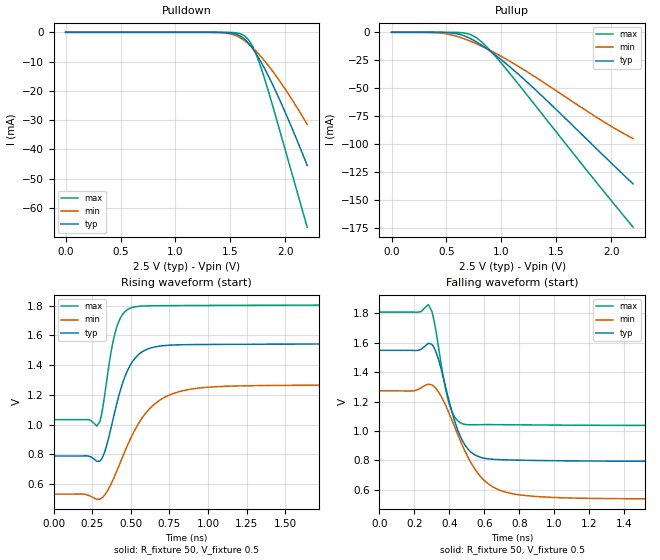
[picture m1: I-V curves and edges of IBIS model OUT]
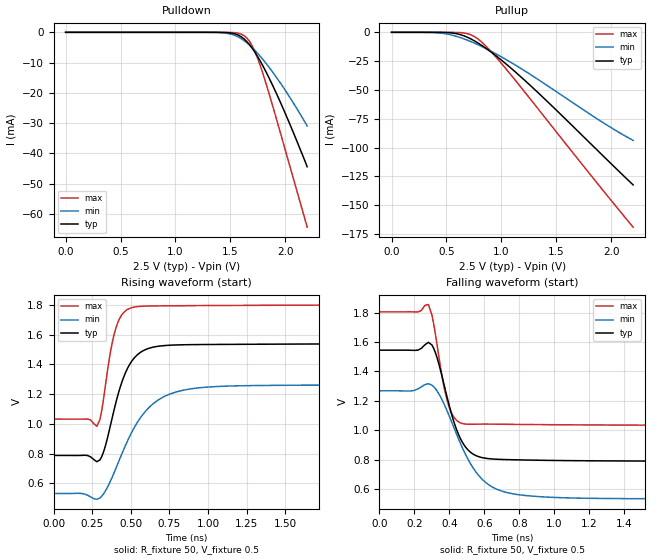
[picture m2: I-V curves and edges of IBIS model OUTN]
|   IBIS File of SG2520EGN D
|   LV-PECL, Vcc=2.5V, fo<=212.5MHz
[IBIS Ver]   3.2
[File Name]   sg2520egn_25v.ibs
[File Rev]   1.0
[Date]   Sep. 2, 2020
[Source]
[Notes]
Created by Minoru Kozaki
[Disclaimer]
Seiko Epson Corporation makes no warranty with respect to the
information contained herein.
[Copyright]
Copyright(C) 2020, Seiko Epson Corporation. All rights reserved.
|   Component
[Component]   SG2520EGN
[Manufacturer]  Seiko Epson Corporation
[Package]
R_pkg   17.7m   NA   NA
L_pkg   235p   NA   NA
C_pkg   208f   NA   NA
[Pin]   signal_name   model_name   R_pin   L_pin   C_pin
1   OE/ST   NC
2   NC   NC
3   GND   GND
4   OUT   OUT   17.7m   235p   208f
5   OUTN   OUTN   10.4m   129p   221f
6   VCC   POWER
[Diff Pin] inv_pin  vdiff  tdelay_typ
4   5   0   0
| Models and submodels in the file (2): OUT (Output_ECL), OUTN (Output_ECL)
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|   Model OUT
[Model]   OUT
Model_type   Output_ECL
Polarity   Non-Inverting
Vref = 0.5
Vmeas = 1.166
Rref = 50
Cref = 0
C_comp   0.5p   0.5p   0.5p
[Temperature Range]   25   105   -40
[Voltage Range]   2.5   2.25   2.75
[Pullup Reference]   2.5   2.25   2.75
[Pulldown Reference]   2.5   2.25   2.75
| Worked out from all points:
|   falling waveform, R_fixture 50, V_fixture 0.5: 20-80 % time 113ps typ, 187ps min, 71.3ps max; typ from 1.55 V to 0.79 V
|   rising waveform, R_fixture 50, V_fixture 0.5: 20-80 % time 131ps typ, 232ps min, 78.7ps max; typ from 0.789 V to 1.55 V
[Pullup]
0V        16.83nA    9.98nA     69.06nA
375mV     -9.189uA   -202.2uA   -2.725uA
550mV     -554.6uA   -2.432mA   -27.27uA
625mV     -1.967mA   -4.553mA   -238.1uA
700mV     -4.74mA    -7.234mA   -1.407mA
750mV     -7.255mA   -9.266mA   -3.486mA
800mV     -10.18mA   -11.46mA   -6.878mA
875mV     -15.15mA   -15.02mA   -13.8mA
950mV     -20.65mA   -18.86mA   -21.92mA
1.225V    -43.68mA   -34.72mA   -54.94mA
1.9V      -107.4mA   -78.03mA   -138.4mA
2.2V      -135.6mA   -95.04mA   -174.3mA
[Pulldown]
0V        16.82nA    9.98nA     69.07nA
1.4V      -18.51uA   -91.51uA   -3.785uA
1.525V    -362.3uA   -815.4uA   -77.68uA
1.625V    -2.189mA   -2.757mA   -1.1mA
1.675V    -4.128mA   -4.268mA   -3.029mA
1.7V      -5.352mA   -5.139mA   -4.597mA
1.725V    -6.722mA   -6.076mA   -6.581mA
1.775V    -9.826mA   -8.123mA   -11.57mA
1.85V     -15.16mA   -11.56mA   -20.58mA
1.95V     -23.12mA   -16.67mA   -33.56mA
2.075V    -33.97mA   -23.75mA   -50.1mA
2.2V      -45.49mA   -31.44mA   -66.58mA
[Falling Waveform]
R_fixture = 50
V_fixture = 0.5
V_fixture_min = 0.25
V_fixture_max = 0.75
0s        1.549V     1.273V     1.809V
220ps     1.548V     1.282V     1.808V
280ps     1.598V     1.318V     1.861V
300ps     1.59V      1.313V     1.815V
330ps     1.516V     1.279V     1.631V
400ps     1.196V     1.116V     1.181V
490ps     902.1mV    859.9mV    1.044V
640ps     807.2mV    624.7mV    1.043V
880ps     798.8mV    554.5mV    1.04V
4ns       789.7mV    533.5mV    1.034V
[Rising Waveform]
R_fixture = 50
V_fixture = 0.5
V_fixture_min = 0.25
V_fixture_max = 0.75
0s        788.8mV    532.3mV    1.033V
280ps     753mV      497.2mV    989.5mV
300ps     754.5mV    498.3mV    1.021V
330ps     813.3mV    524.8mV    1.19V
370ps     968mV      595.1mV    1.474V
410ps     1.144V     688.7mV    1.659V
530ps     1.45V      970.8mV    1.793V
700ps     1.53V      1.172V     1.8V
980ps     1.539V     1.25V      1.802V
4ns       1.547V     1.271V     1.808V
[Ramp]
R_load = 50
dV/dt_r   0.45322/130.05p   0.44158/230.87p   0.46303/78.13p
dV/dt_f   0.45322/112.19p   0.44158/186.60p   0.46303/70.64p
|   Model OUTN
[Model]   OUTN
Model_type   Output_ECL
Polarity   Inverting
Vref = 0.5
Vmeas = 1.166
Rref = 50
Cref = 0
C_comp   0.5p   0.5p   0.5p
[Temperature Range]   25   105   -40
[Voltage Range]   2.5   2.25   2.75
[Pullup Reference]   2.5   2.25   2.75
[Pulldown Reference]   2.5   2.25   2.75
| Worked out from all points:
|   falling waveform, R_fixture 50, V_fixture 0.5: 20-80 % time 113ps typ, 188ps min, 70.7ps max; typ from 1.54 V to 0.789 V
|   rising waveform, R_fixture 50, V_fixture 0.5: 20-80 % time 131ps typ, 233ps min, 78.9ps max; typ from 0.788 V to 1.54 V
[Pullup]
0V        16.82nA    9.979nA    69.06nA
375mV     -9.188uA   -202uA     -2.725uA
550mV     -553.1uA   -2.417mA   -27.26uA
625mV     -1.953mA   -4.515mA   -237.7uA
700mV     -4.684mA   -7.162mA   -1.396mA
750mV     -7.154mA   -9.165mA   -3.437mA
800mV     -10.02mA   -11.33mA   -6.739mA
875mV     -14.88mA   -14.83mA   -13.44mA
950mV     -20.24mA   -18.61mA   -21.29mA
1.25V     -44.86mA   -35.68mA   -56.2mA
1.9V      -104.7mA   -76.73mA   -134mA
2.2V      -132.3mA   -93.71mA   -169mA
[Pulldown]
0V        16.82nA    9.978nA    69.06nA
1.4V      -18.51uA   -91.47uA   -3.785uA
1.525V    -361.6uA   -812.9uA   -77.64uA
1.625V    -2.171mA   -2.738mA   -1.093mA
1.675V    -4.08mA    -4.232mA   -2.987mA
1.7V      -5.281mA   -5.091mA   -4.514mA
1.725V    -6.624mA   -6.016mA   -6.436mA
1.775V    -9.661mA   -8.034mA   -11.25mA
1.85V     -14.87mA   -11.41mA   -19.92mA
1.95V     -22.63mA   -16.44mA   -32.45mA
2.075V    -33.19mA   -23.39mA   -48.41mA
2.2V      -44.4mA    -30.93mA   -64.35mA
[Falling Waveform]
R_fixture = 50
V_fixture = 0.5
V_fixture_min = 0.25
V_fixture_max = 0.75
0s        1.545V     1.269V     1.805V
220ps     1.545V     1.281V     1.804V
280ps     1.598V     1.317V     1.855V
320ps     1.528V     1.284V     1.655V
390ps     1.212V     1.124V     1.192V
430ps     1.043V     1.007V     1.083V
480ps     908.8mV    867.8mV    1.045V
630ps     808mV      627.6mV    1.043V
880ps     798.4mV    553.8mV    1.04V
4ns       788.6mV    532.6mV    1.033V
[Rising Waveform]
R_fixture = 50
V_fixture = 0.5
V_fixture_min = 0.25
V_fixture_max = 0.75
0s        787.7mV    531.3mV    1.032V
280ps     745.4mV    492.2mV    983.7mV
300ps     757.3mV    501.6mV    1.028V
330ps     831.8mV    539.1mV    1.214V
400ps     1.128V     691.3mV    1.633V
450ps     1.303V     817.1mV    1.745V
520ps     1.441V     970.2mV    1.786V
700ps     1.525V     1.175V     1.794V
980ps     1.534V     1.246V     1.796V
4ns       1.543V     1.267V     1.803V
[Ramp]
R_load = 50
dV/dt_r   0.45129/130.71p   0.43982/232.32p   0.46093/78.16p
dV/dt_f   0.45129/112.18p   0.43982/187.05p   0.46093/70.32p
